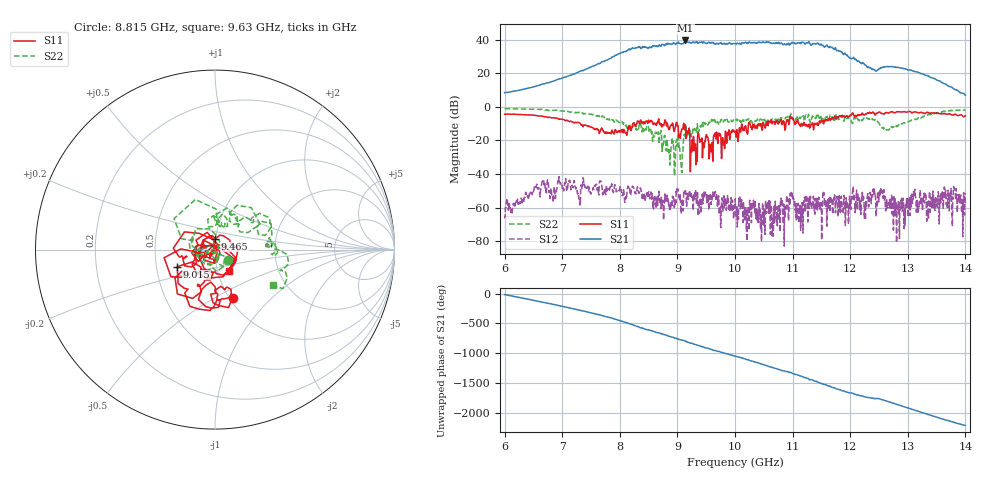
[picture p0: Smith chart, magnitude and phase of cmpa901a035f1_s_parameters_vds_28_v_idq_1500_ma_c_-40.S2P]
!Keysight Technologies,E5071C,MY46110325,B.14.03
!Date: Wed Mar 10 09:54:20 2021
!Data & Calibration Information:
!Freq	S11:SOLT2(ON)	S21:SOLT2(ON)	S12:SOLT2(ON)	S22:SOLT2(ON)
!PortZ  Port1:50+j0  Port2:50+j0
!Above PortZ is port z conversion or system Z0 setting when saving the data.
!When reading, reference impedance value at option line is always used.
# Hz S dB R 50
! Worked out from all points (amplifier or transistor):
!   1601 points, 6 GHz to 14 GHz, reference 50 ohm
!   highest |S21| = 39.5 dB at 9.14 GHz (marker M1)
!   |S21| within 3 dB of that: 8.783 GHz to 11.51 GHz (2.732 GHz wide, 26.9 % of centre)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
!   unconditionally stable (mu >= 1): start of sweep to end of sweep
!   at 7.33 GHz: K = 5.20, MAG = 24.0 dB, |S12| = -46.9 dB
!   at 10 GHz: K = 4.84, MAG = 38.5 dB, |S12| = -58.9 dB
!   at 14 GHz: K = 21.59, MAG = 12.7 dB, |S12| = -51.4 dB
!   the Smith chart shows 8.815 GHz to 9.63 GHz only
!   S11 on the Smith chart (normalised r, x): 8.815 GHz: 1.04, -0.60; 9.015 GHz: 0.64, -0.13; 9.465 GHz: 0.99, +0.12; 9.63 GHz: 1.13, -0.27
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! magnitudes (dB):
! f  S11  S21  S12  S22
! 6 GHz  -4.5  8.4  -65.0  -1.1
! 6.67 GHz  -5.7  13.6  -43.8  -1.7
! 7.335 GHz  -10.9  21.3  -47.7  -3.7
! 8.67 GHz  -7.9  35.9  -53.6  -15.1
! 8.815 GHz  -10.9  37.0  -55.3  -20.5
! 9.015 GHz  -12.7  38.5  -49.0  -16.0
! 9.065 GHz  -14.9  37.4  -63.6  -35.1
! 9.14 GHz  -10.8  39.5  -49.1  -10.9
! 9.26 GHz  -20.7  38.2  -54.3  -16.3
! 9.465 GHz  -24.3  38.4  -54.0  -9.6
! 9.63 GHz  -17.1  37.7  -51.1  -8.4
! 10 GHz  -15.2  37.6  -58.9  -8.1
! 10.21 GHz  -14.5  38.0  -63.0  -7.9
! 10.32 GHz  -12.1  38.0  -55.5  -9.3
! 10.48 GHz  -11.5  38.5  -57.1  -8.3
! 10.98 GHz  -7.0  37.9  -53.1  -5.9
! 11.14 GHz  -10.6  37.7  -58.8  -6.3
! 11.34 GHz  -10.6  37.1  -58.3  -6.6
! 11.94 GHz  -5.2  30.5  -58.9  -7.0
! 12.55 GHz  -4.0  23.4  -51.8  -12.6
! 12.67 GHz  -3.7  23.8  -58.2  -13.6
! 14 GHz  -5.3  6.8  -51.4  -1.9
